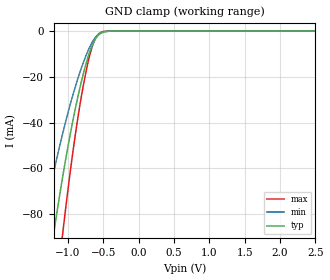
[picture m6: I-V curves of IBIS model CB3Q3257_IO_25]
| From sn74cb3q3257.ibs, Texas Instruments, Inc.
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[Model]   CB3Q3257_IO_25
Model_type  Terminator
| variable   typ   min   max
C_comp   7.11pF   5.12pF   11.67pF
| C_tri-state   7.11pF   5.12pF   11.67pF
[Temperature Range]   40   100   -40
| Ambient temperature   25   85   -40
[Voltage range]   2.5   2.3   2.7
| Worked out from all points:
|   GND clamp passes 1 mA (typ) near -0.54 V on its own axis
[GND Clamp]
| CB3Q3257_IO_25
|   Voltage   I(typ)   I(min)   I(max)
-5.5V     -1.394A    -1.081A    -1.727A
-1.38V    -127.2mA   -88.48mA   -178.7mA
-1.355V   -121.5mA   -84.53mA   -170.8mA
-1.2V     -88.06mA   -61.43mA   -123.6mA
-1.08V    -64.62mA   -45.4mA    -89.91mA
-1.06V    -60.96mA   -42.89mA   -84.6mA
-890mV    -33mA      -23.73mA   -44.03mA
-775mV    -17.73mA   -13.11mA   -22.5mA
-660mV    -6.502mA   -5.038mA   -7.071mA
-555mV    -1.372mA   -1.126mA   -930.6uA
-355mV    -9.503uA   -13.95uA   -1.12uA
2.5V      187.7pA    872.9pA    23.66pA
